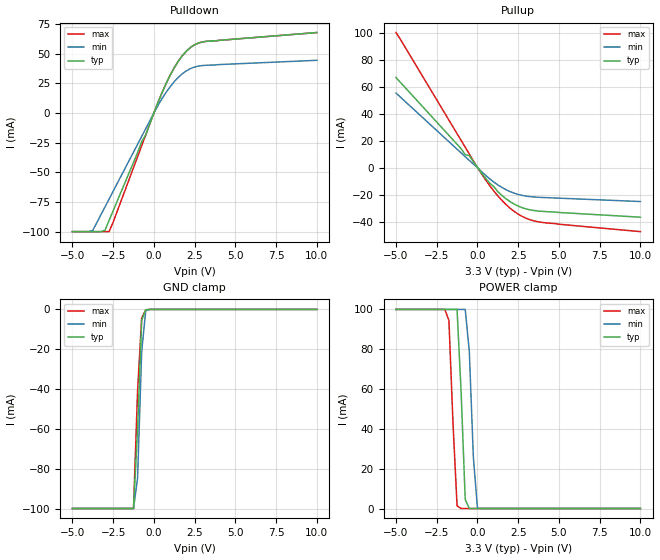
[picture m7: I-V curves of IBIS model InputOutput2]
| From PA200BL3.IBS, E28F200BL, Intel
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|**********************Input Output Model 2*************************
[Model]   InputOutput2
Model_type   I/O
|   Model for DQ[15] pin.
Vinl = 0.8V
Vinh = 2.0V
|Variable   Typ   Min   Max
C_comp   9.61p   NA   11.6p
[Voltage Range]   3.3V   3.0V   3.6V
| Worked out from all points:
|   slope of the pulldown table from 0 to 0.495 V, typ, clamps not added: 29.2 ohm
|   slope of the pullup table from 0 to 0.495 V, typ, clamps not added: 63 ohm
|   GND clamp passes 1 mA (typ) near -0.54 V on its own axis
|   POWER clamp passes 1 mA (typ) near -0.55 V on its own axis
[Pulldown]
| [Pullup] and [Pulldown] IV curves include only the current through
| the channels of output driver transistors when outputs are enabled
| with OE# = VIL.  Although the output driver transistors have np and
| pn diodes inherently created by CMOS IC fabrication between the
| drain and bulk of n-channel and p-channel CMOS transistors,
| the current through these junction diodes is not included in
| [Pullup] or [Pulldown].  Instead that drain/bulk diode current is
| included in the [POWER_clamp] or [GND_clamp] sections, which are
| not dependent on the state of OE# or output data value.
|Voltage   I(typ)   I(min)   I(max)
-5V       -100mA     -100mA     -100mA
-3.75V    -100mA     -98.99mA   -100mA
-3V       -98.8mA    -79.19mA   -100mA
-2.75V    -90.63mA   -72.59mA   -100mA
-750mV    -24.2mA    -19.79mA   -27.65mA
-500mV    -18.49mA   -13.19mA   -18.47mA
500mV     17.12mA    12.09mA    17.12mA
1V        31.88mA    22.18mA    31.88mA
1.5V      43.68mA    30.06mA    43.68mA
2.25V     55.27mA    37.45mA    55.27mA
3.25V     60.42mA    40.25mA    60.42mA
10V       67.8mA     44.4mA     67.8mA
[GND_clamp]
| [POWER_clamp] and [GND_clamp] IV curves describe ESD protection
| circuits PLUS some np and pn diodes which exist between the
| drain and bulk of n-channel and p-channel CMOS transistors.
| These drain/bulk diodes are inherent in CMOS IC fabrication,
| and are visible on the node of the I/O pin at all times.
| Even the drain/bulk diodes of output driver [Pullup] and [Powerdown]
| transistors are included in [POWER_clamp] or [GND_clamp], because
| these diodes contribute to I/O pin current even when the
| chip outputs are tristated by OE# = VIH.
| For example, when V forced on the I/O pin is large, we are
| forward biasing the pn diode at the drain/bulk interface in the
| p-channel pullup transistor.  Similarly, when V forced on the
| I/O pin is sufficiently negative with respect to the substrate
| ground, we are forward biasing the np diode at the drain/bulk
| interface in the n-channel pulldown transistor.  The effects
| of these diodes are included in [POWER_clamp] or [GND_clamp].
|Voltage   I(typ)   I(min)   I(max)
-5V       -99.85mA   -99.85mA   -99.85mA
-1.25V    -99.85mA   -99.85mA   -99.85mA
-1V       -60mA      -84.53mA   -40.79mA
-750mV    -5.562mA   -21.29mA   -4.395mA
-500mV    -191.4uA   -722.8uA   -214.3uA
-250mV    -32.36nA   -2.075uA   -15.38nA
10V       0A         0A         0A
[Pullup]
| (Voltages for [Pullup] and [POWER_clamp] are specified with
| negative respect to Vcc.  Reference the IBIS documentation
| for more information regarding Vtable = Vcc - Voutput.
| This method keeps -Vds constant for the values in all three
| columns across a line of the table.
| [Pullup] and [Pulldown] IV curves include only the current through
| the channels of output driver transistors when outputs are enabled
| with OE# = VIL.  Although the output driver transistors have np and
| pn diodes inherently created by CMOS IC fabrication between the
| drain and bulk of n-channel and p-channel CMOS transistors,
| the current through these junction diodes is not included in
| [Pullup] or [Pulldown].  Instead that drain/bulk diode current is
| included in the [POWER_clamp] or [GND_clamp] sections, which are
| not dependent on the state of OE# or output data value.
|Voltage  I(typ)   I(min)   I(max)
-5V       66.7mA     55.2mA     100mA
-1V       13.9mA     10.8mA     20.07mA
-750mV    9.488mA    8.025mA    15.05mA
-500mV    8.818mA    5.25mA     10.04mA
250mV     -4.084mA   -3.031mA   -4.666mA
750mV     -11.54mA   -8.388mA   -13.34mA
1V        -14.07mA   -10.73mA   -17.29mA
1.25V     -17.91mA   -12.86mA   -20.98mA
2V        -25.25mA   -17.83mA   -30.11mA
2.75V     -29.8mA    -20.67mA   -36.27mA
3.75V     -32.34mA   -22.03mA   -40.27mA
10V       -36.8mA    -25.2mA    -47.5mA
[POWER_clamp]
| (Voltages for [Pullup] and [POWER_clamp] are specified with
| negative respect to Vcc.  Reference the IBIS documentation
| for more information regarding Vtable = Vcc - Voutput.
| This method keeps -Vds constant for the values in all three
| columns across a line of the table.
| [POWER_clamp] and [GND_clamp] IV curves describe ESD protection
| circuits PLUS some np and pn diodes which exist between the
| drain and bulk of n-channel and p-channel CMOS transistors.
| These drain/bulk diodes are inherent in CMOS IC fabrication,
| and are visible on the node of the I/O pin at all times.
| Even the drain/bulk diodes of output driver [Pullup] and [Powerdown]
| transistors are included in [POWER_clamp] or [GND_clamp], because
| these diodes contribute to I/O pin current even when the
| chip outputs are tristated by OE# = VIH.
| For example, when V forced on the I/O pin is large, we are
| forward biasing the pn diode at the drain/bulk interface in the
| p-channel pullup transistor.  Similarly, when V forced on the
| I/O pin is sufficiently negative with respect to the substrate
| ground, we are forward biasing the np diode at the drain/bulk
| interface in the n-channel pulldown transistor.  The effects
| of these diodes are included in [POWER_clamp] or [GND_clamp].
|Voltage I(typ)   I(min)   I(max)
-5V       100mA      100mA      100mA
-2V       100mA      100mA      100mA
-1.75V    100mA      100mA      94.44mA
-1.5V     100mA      100mA      42.84mA
-1.25V    100mA      100mA      1.343mA
-1V       58.11mA    100mA      40.86nA
-750mV    4.582mA    100mA      0A
-500mV    543.5nA    79.07mA    0A
-250mV    0A         25.67mA    0A
0V        0A         242.8uA    0A
10V       0A         0A         0A
[Ramp]
| The RY/BY# Ramp information is not provided for this device.  The table
| below is for the compatibility with some IBIS parsers.
| Variable   typ   min   max
 dV/dt_r   0V/0ns   0V/0ns   0V/0ns
 dV/dt_f   0V/0ns   0V/0ns   0V/0ns
